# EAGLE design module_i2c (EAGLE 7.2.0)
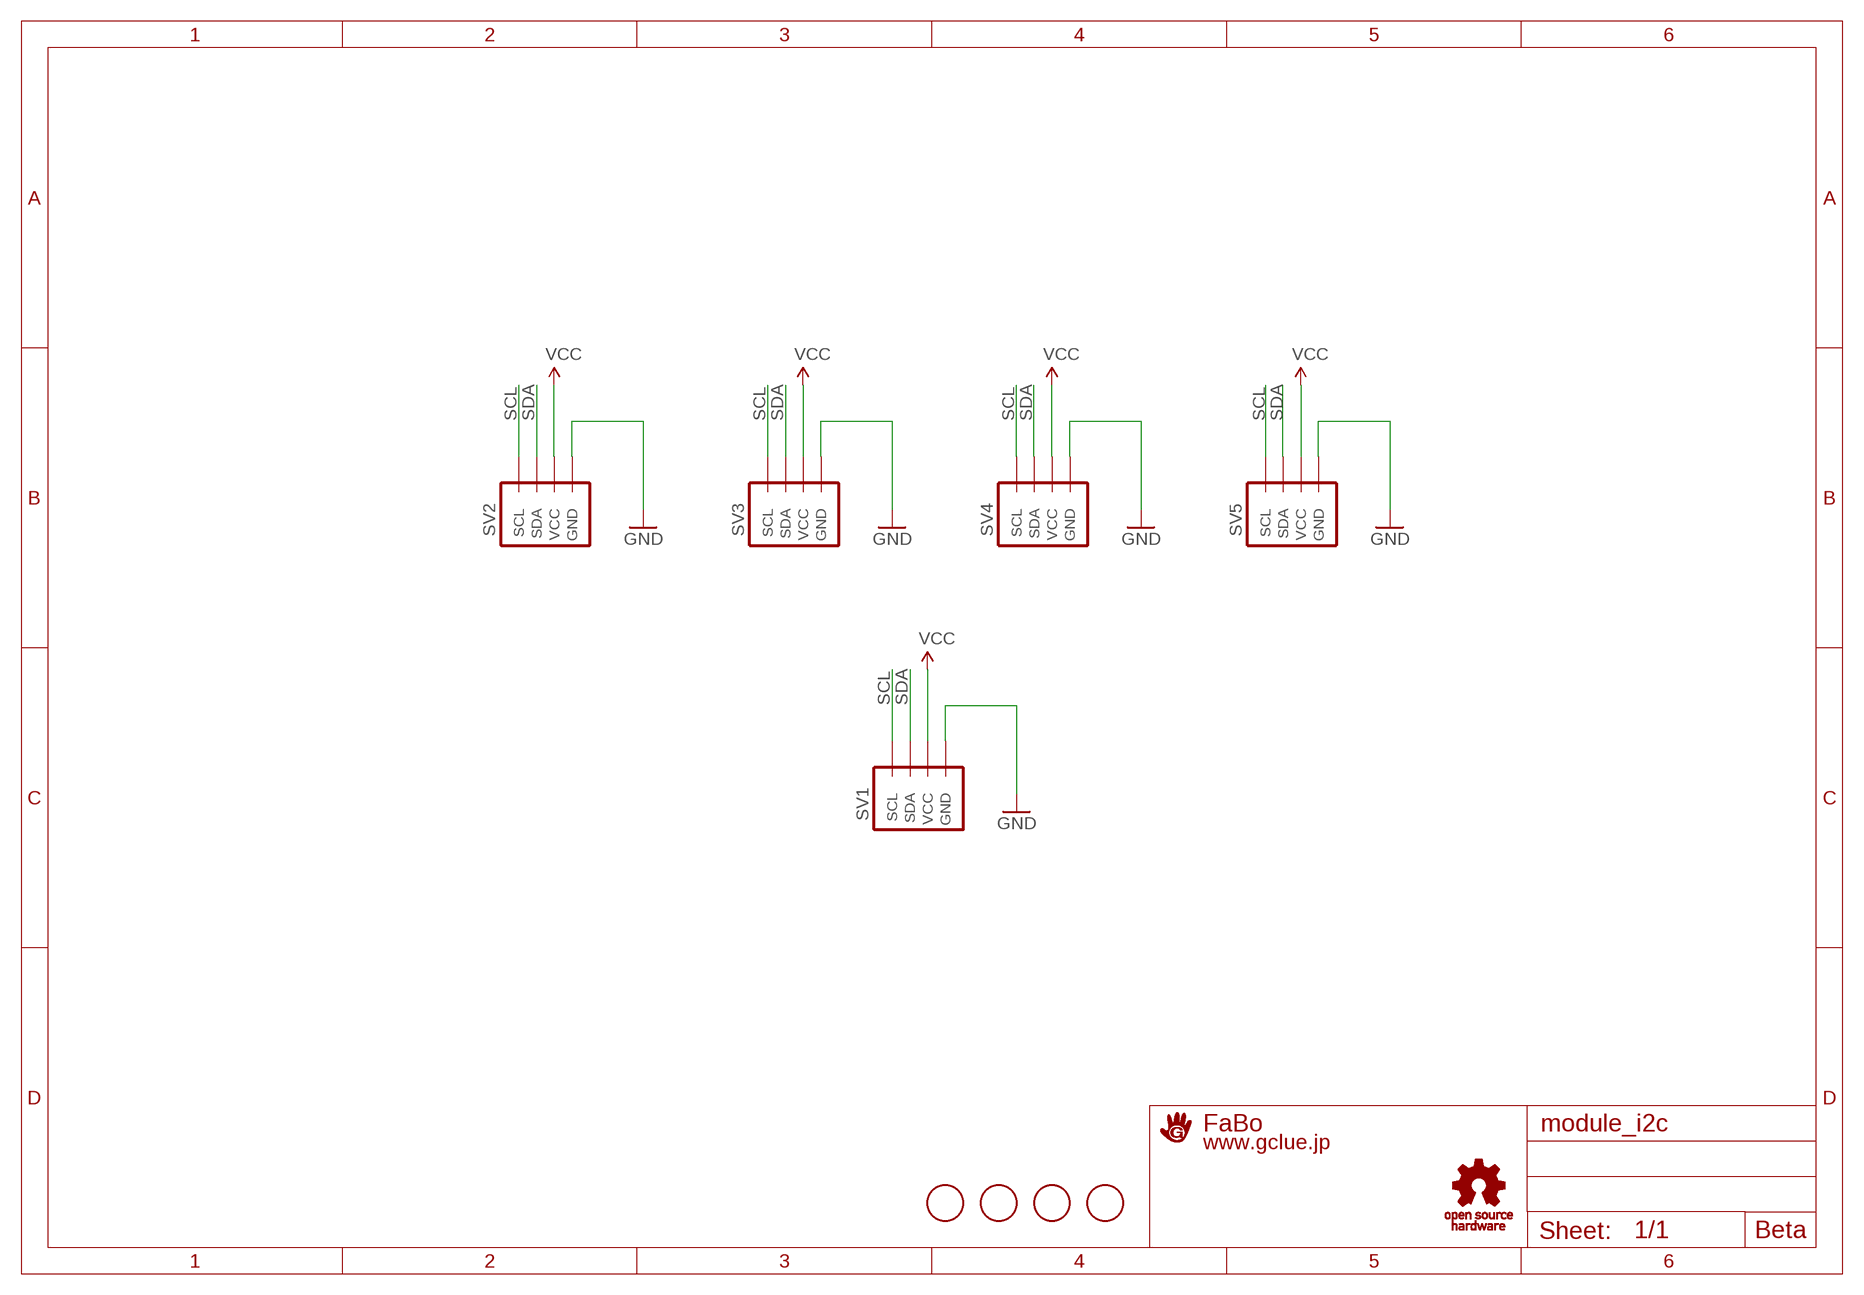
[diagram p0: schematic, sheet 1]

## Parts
SV1  BRICK_I2C_CONNECTOR  [BRICK_I2C_CONNECTOR]
SV2  BRICK_I2C_CONNECTOR  [BRICK_I2C_CONNECTOR]
SV3  BRICK_I2C_CONNECTOR  [BRICK_I2C_CONNECTOR]
SV4  BRICK_I2C_CONNECTOR  [BRICK_I2C_CONNECTOR]
SV5  BRICK_I2C_CONNECTOR  [BRICK_I2C_CONNECTOR]
U$7  SCREW-PAD-3MM  [SCREWPAD_3MM]
U$8  SCREW-PAD-3MM  [SCREWPAD_3MM]
U$9  SCREW-PAD-3MM  [SCREWPAD_3MM]
U$10  SCREW-PAD-3MM  [SCREWPAD_3MM]
U$11  LOGO_OSHW_T-M  [LOGO_OSHW_T_M]
U$12  LOGO_GCLUE-M  [LOGO_GCLUE_M]

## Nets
GND [PWR]: SV1.GND SV2.GND SV3.GND SV4.GND SV5.GND
SCL: SV1.SCL SV2.SCL SV3.SCL SV4.SCL SV5.SCL
SDA: SV1.SDA SV2.SDA SV3.SDA SV4.SDA SV5.SDA
VCC [PWR]: SV1.VCC SV2.VCC SV3.VCC SV4.VCC SV5.VCC

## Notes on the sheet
- Beta

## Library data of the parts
SV1-SV5 = gclue:BRICK_I2C_CONNECTOR: Brick Connector female for OUT/IN Shield
U$7-U$10 = gclue:SCREW-PAD
U$11 = gclue:LOGO_OSHW_T
U$12 = gclue:LOGO_GCLUE

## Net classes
0 default: width 0.406 mm
1 PWR: width 0.61 mm

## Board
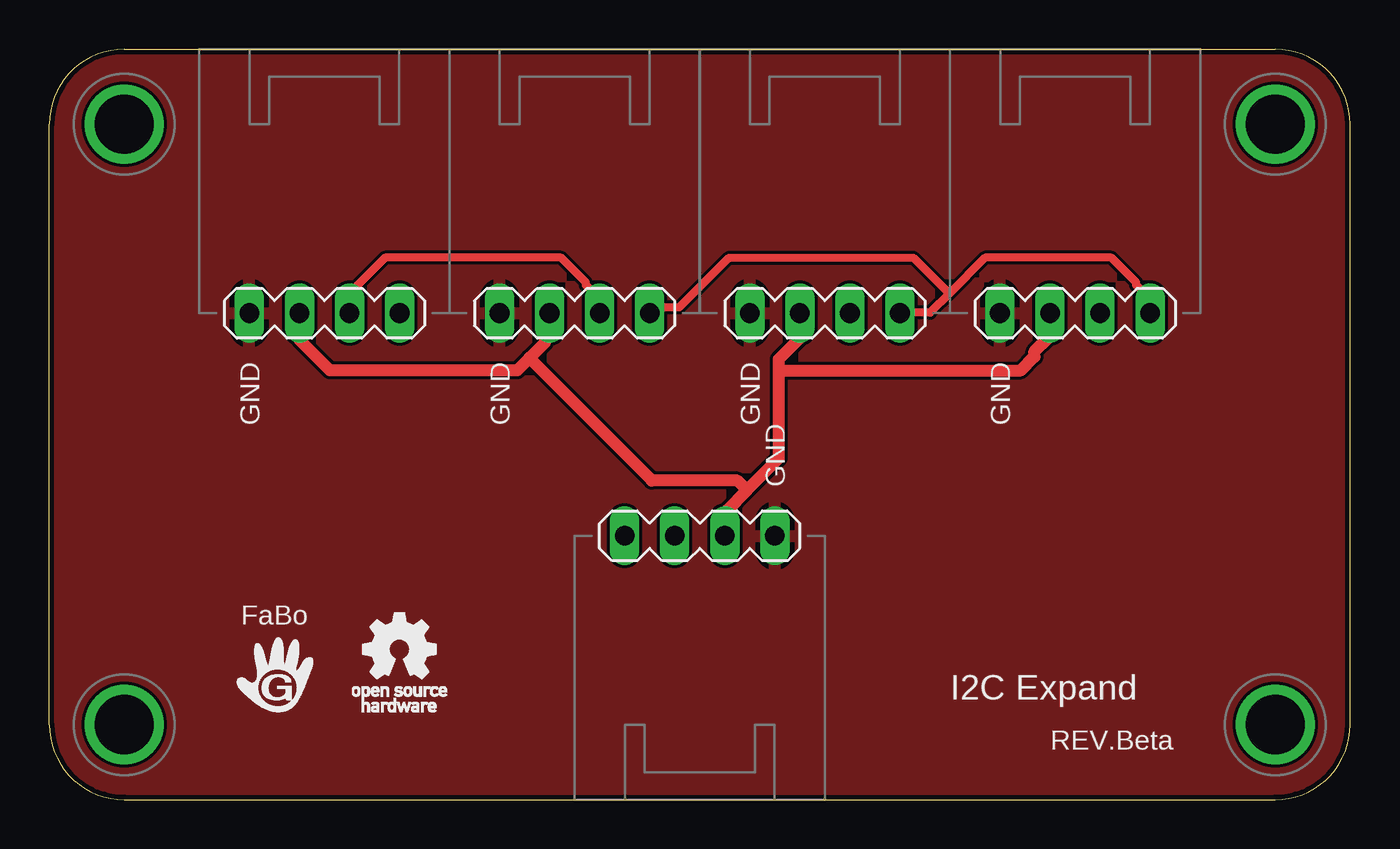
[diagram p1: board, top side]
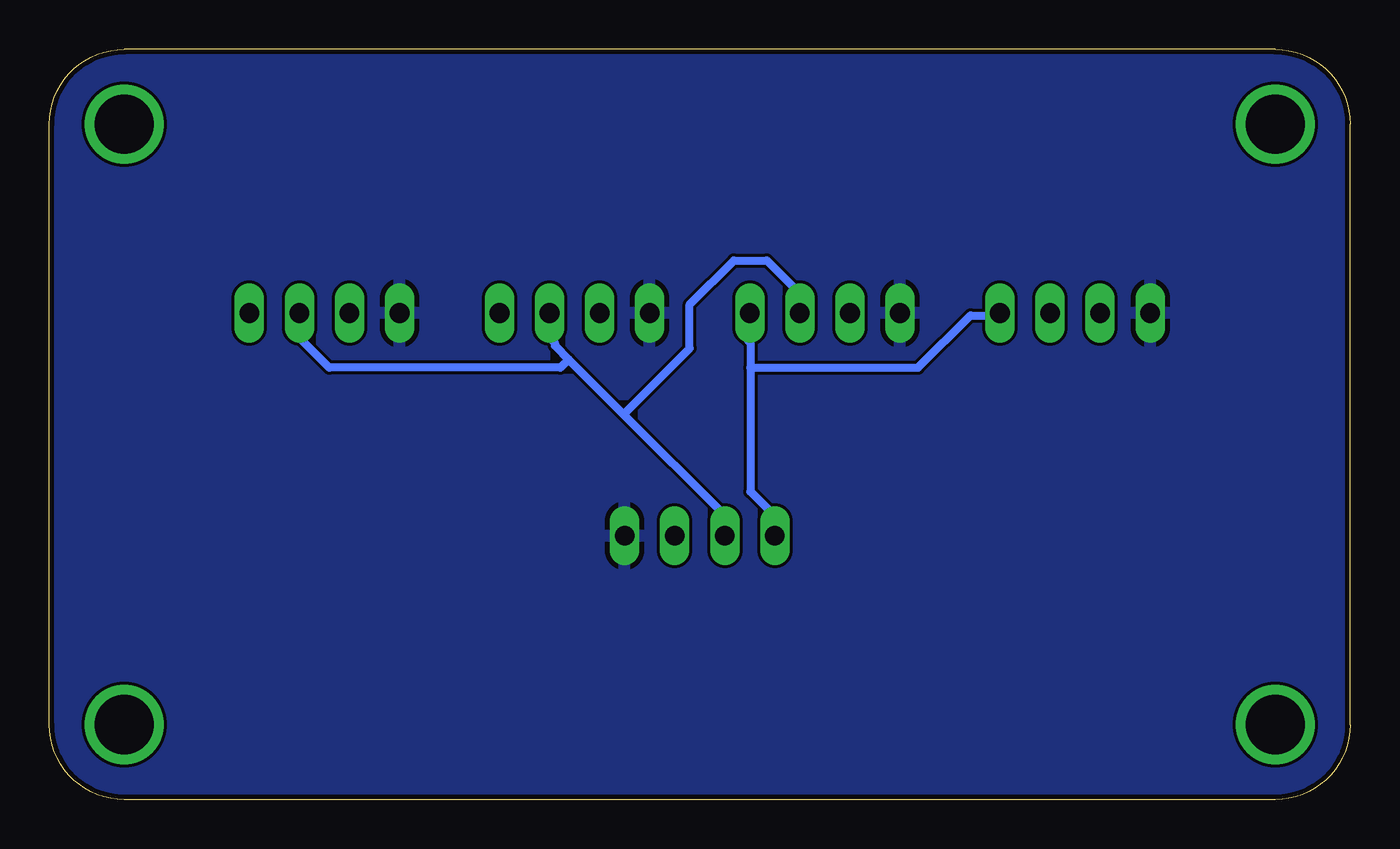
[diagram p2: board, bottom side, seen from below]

Size 66.04 x 38.1 mm. Coordinates in mm from the lower left corner, seen from the top.
Outline: 3.81,0 62.23,0 arc90 66.04,3.81 66.04,34.29 arc90 62.23,38.1 3.81,38.1 arc90 0,34.29 0,3.81 arc90 3.81,0
Copper layers (1*16): Top 0.035mm / dielectric 1.5mm / Bottom 0.035mm
Design rules "Elecrow_2-layer_eagle_rule": minimum track width 6mil, minimum drill 12mil, track to track 6mil, track to pad 6mil, pad to pad 6mil, via to via 6mil, smd to smd 0mil, copper to edge 10mil, drill to drill 10mil, minimum pad ring 10mil, minimum via ring 6mil, stop-mask expansion 2mil, vias tented up to drill 100mil, thermal gap 10mil

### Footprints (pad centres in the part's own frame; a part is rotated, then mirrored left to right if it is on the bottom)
BRICK_I2C_CONNECTOR = drill 1 long: GND -3.81,0; SCL 3.81,0; SDA 1.27,0; VCC -1.27,0
SCREWPAD_3MM = drill 3 pad 3.81: 1 0,0

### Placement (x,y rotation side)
SV1  33.02,13.4 180 top
SV2  13.97,24.7 0 top
SV3  26.67,24.7 0 top
SV4  39.37,24.7 0 top
SV5  52.07,24.7 0 top
U$7  3.81,3.81 0 top
U$8  3.81,34.29 0 top
U$9  62.23,34.29 0 top
U$10  62.23,3.81 0 top
U$11  17.78,7.62 0 top
U$12  11.43,6.35 0 top

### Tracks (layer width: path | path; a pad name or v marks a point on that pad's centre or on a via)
GND
  pour Top: -1.27,-1.27 67.31,-1.27 67.31,39.37 -1.27,39.37
  pour Bottom: -1.27,-1.27 67.31,-1.27 67.31,39.37 -1.27,39.37
SCL
  Top 0.406: 45.68,25.7 47.5,27.52 53.92,27.52 55.18,26.26 55.18,26.12 55.88,25.43 SV5.SCL | 45.68,25.7 44.7,24.73 43.31,24.73 SV4.SCL | 45.68,25.7 43.87,27.52 34.51,27.52 31.99,25.01 30.87,25.01 30.59,24.73 SV3.SCL
  Bottom 0.406: 30.45,21.93 30.45,23.19 30.59,23.33 30.59,24.59 SV3.SCL | 30.45,21.93 30.45,15.65 29.34,14.53 29.34,13.41 SV1.SCL | 30.45,21.93 21.93,21.93 19.28,24.59 17.88,24.59 SV2.SCL
SDA
  Top 0.406: SV3.SDA 27.94,25.43 27.24,26.12 27.24,26.26 25.98,27.52 17.04,27.52 15.37,25.84 15.37,24.73 SV2.SDA
  Bottom 0.406: 39.67,22.35 40.37,23.05 40.37,23.19 40.51,23.33 40.51,24.59 SV4.SDA | 39.67,22.35 36.88,19.56 | 36.88,19.56 31.85,14.53 31.85,13.41 SV1.SDA | 39.67,22.35 40.09,21.93 51.83,21.93 53.23,23.33 53.23,24.59 SV5.SDA | SV3.SDA 27.94,25.7 29.62,27.38 31.29,27.38 33.53,25.15 33.53,22.91 36.88,19.56
VCC
  Top 0.61: 24.38,22.42 25.15,23.19 25.15,23.33 25.29,23.47 25.29,24.59 SV3.VCC | 24.38,22.42 23.75,21.79 14.25,21.79 12.71,23.33 12.71,24.59 SV2.VCC | 35.41,15.72 37.02,17.32 37.02,21.79 | 35.41,15.72 34.37,14.67 34.37,13.41 SV1.VCC | 37.02,21.79 37.02,22.35 38.14,23.47 38.14,24.59 SV4.VCC | 37.02,21.79 49.31,21.79 50.01,22.49 50.01,22.77 50.71,23.47 50.71,24.59 SV5.VCC | 24.38,22.42 30.59,16.2 34.92,16.2 35.41,15.72

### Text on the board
tPlace: GND | GND | GND | GND | GND | FaBo | I2C Expand | REV.Beta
